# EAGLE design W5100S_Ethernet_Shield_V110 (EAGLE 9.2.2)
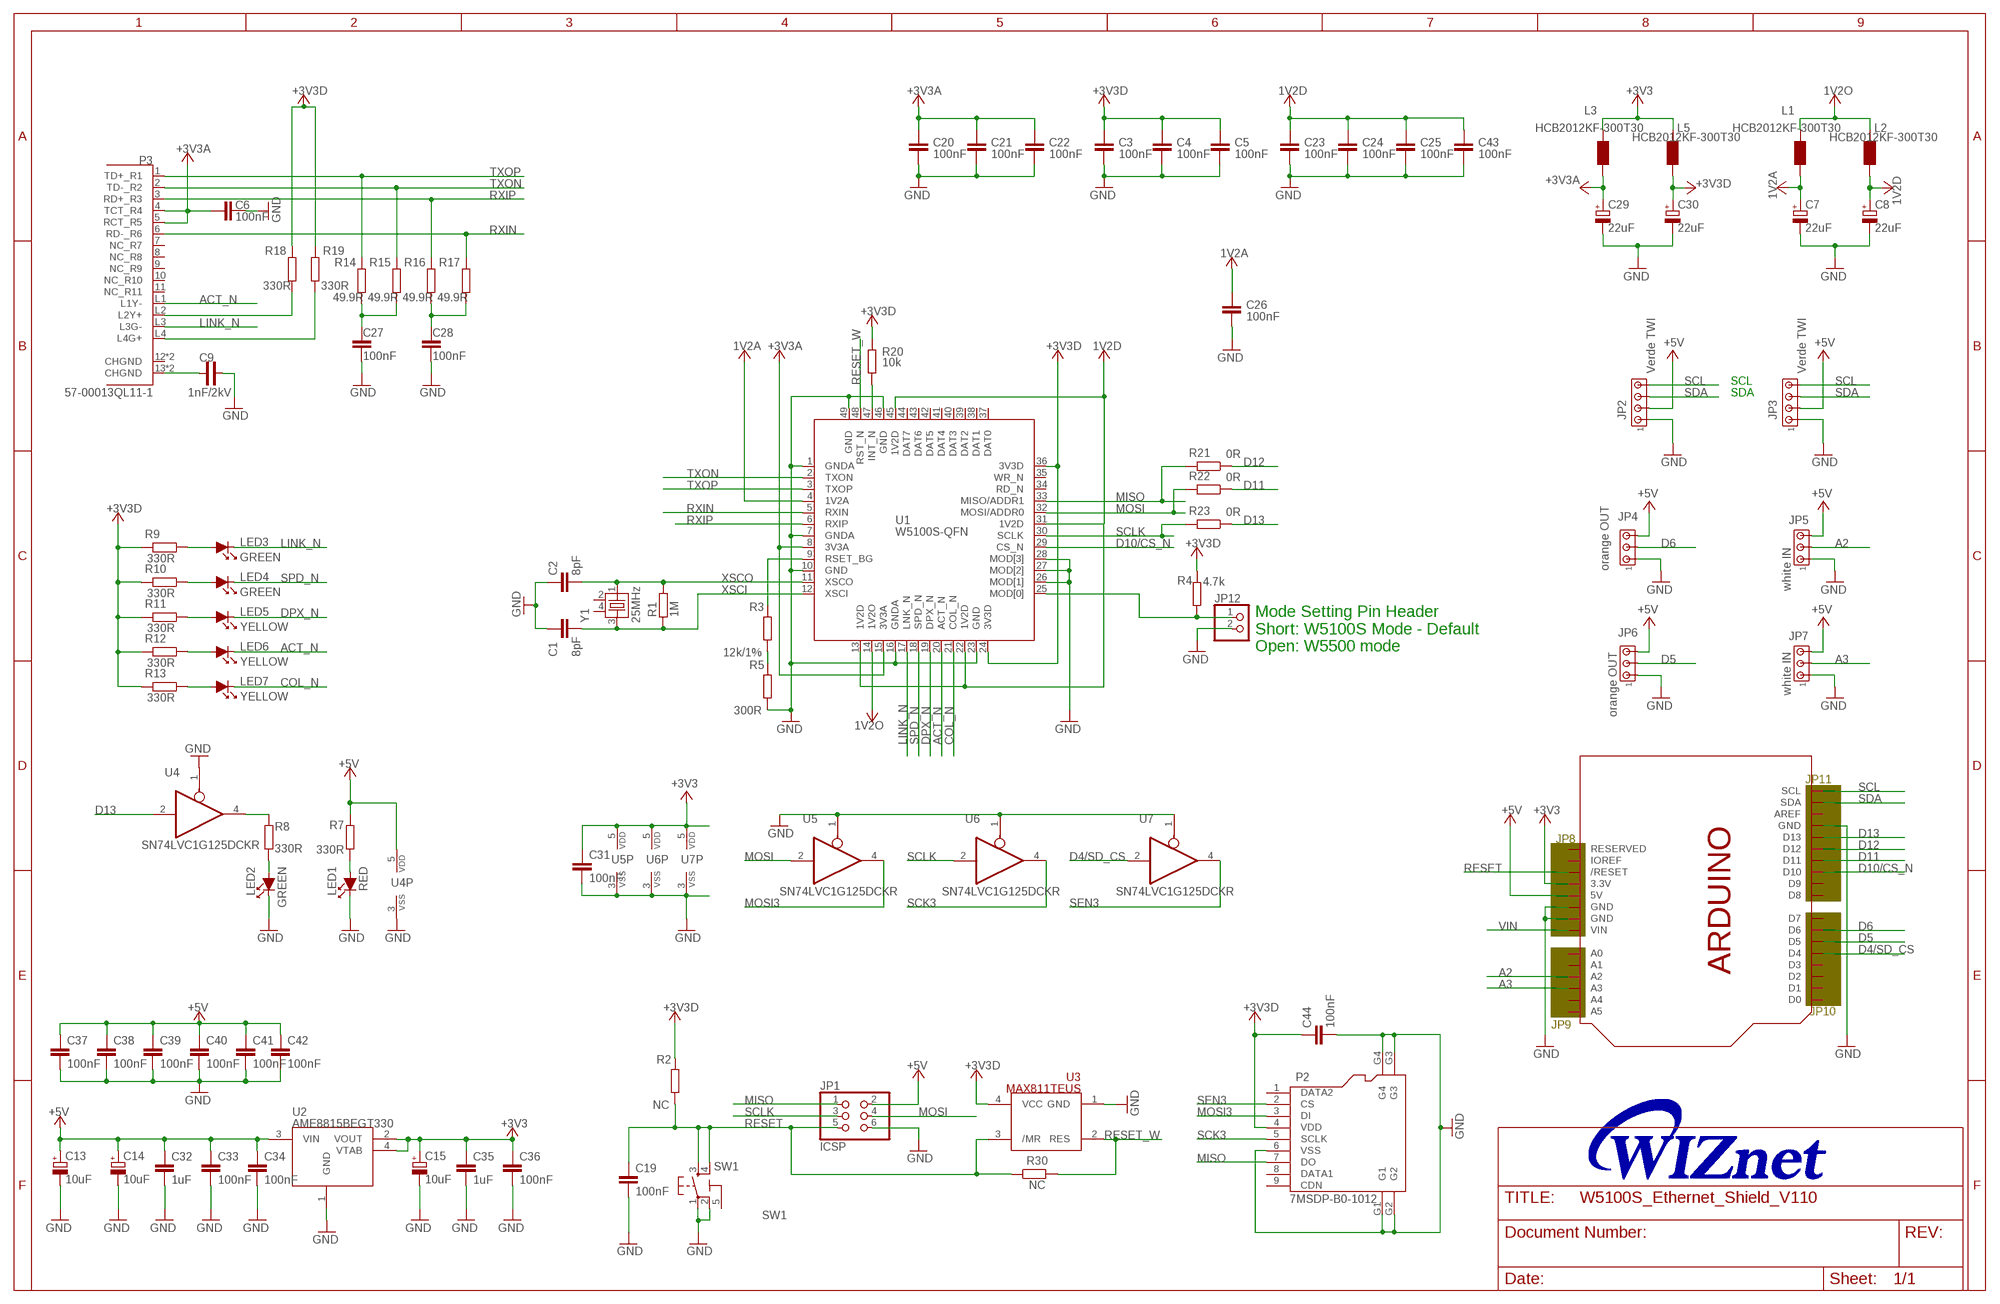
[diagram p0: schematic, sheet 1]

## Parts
C1  8pF  C-EU0603-RND  [C0603-ROUND]
C2  8pF  C-EU0603-RND  [C0603-ROUND]
C3  100nF  C-EU0603-RND  [C0603-ROUND]
C4  100nF  C-EU0603-RND  [C0603-ROUND]
C5  100nF  C-EU0603-RND  [C0603-ROUND]
C6  100nF  0142_10NF_0603  [C0603-ROUND@1]
C7  22uF  0474_TAJA475M016RNJ  [SMC_A]
C8  22uF  0474_TAJA475M016RNJ  [SMC_A]
C9  1nF/2kV  C-4520  [C-4520]
C13  10uF  0474_TAJA475M016RNJ  [SMC_A]
C14  10uF  0474_TAJA475M016RNJ  [SMC_A]
C15  10uF  0474_TAJA475M016RNJ  [SMC_A]
C19  100nF  0142_10NF_0603  [C0603-ROUND@1]
C20  100nF  C-EU0603-RND  [C0603-ROUND]
C21  100nF  C-EU0603-RND  [C0603-ROUND]
C22  100nF  C-EU0603-RND  [C0603-ROUND]
C23  100nF  C-EU0603-RND  [C0603-ROUND]
C24  100nF  C-EU0603-RND  [C0603-ROUND]
C25  100nF  C-EU0603-RND  [C0603-ROUND]
C26  100nF  C-EU0603-RND  [C0603-ROUND]
C27  100nF  0142_10NF_0603  [C0603-ROUND@1]
C28  100nF  0142_10NF_0603  [C0603-ROUND@1]
C29  22uF  0474_TAJA475M016RNJ  [SMC_A]
C30  22uF  0474_TAJA475M016RNJ  [SMC_A]
C31  100nF  0006_1UF_0603/GRM188R61E105KA12D  [C0603-ROUND]
C32  1uF  0142_10NF_0603  [C0603-ROUND@1]
C33  100nF  0142_10NF_0603  [C0603-ROUND@1]
C34  100nF  0142_10NF_0603  [C0603-ROUND@1]
C35  1uF  0142_10NF_0603  [C0603-ROUND@1]
C36  100nF  0142_10NF_0603  [C0603-ROUND@1]
C37  100nF  0142_10NF_0603  [C0603-ROUND@1]
C38  100nF  0142_10NF_0603  [C0603-ROUND@1]
C39  100nF  0142_10NF_0603  [C0603-ROUND@1]
C40  100nF  0142_10NF_0603  [C0603-ROUND@1]
C41  100nF  0142_10NF_0603  [C0603-ROUND@1]
C42  100nF  0142_10NF_0603  [C0603-ROUND@1]
C43  100nF  C-EU0603-RND  [C0603-ROUND]
C44  100nF  0006_1UF_0603/GRM188R61E105KA12D  [C0603-ROUND]
JP1  ICSP  0114_PH254-203DF118A00V  [2X03]
JP2  Verde TWI  1693_WA254-04S-632  [10X04MTA]
JP3  Verde TWI  1693_WA254-04S-632  [10X04MTA]
JP4  orange OUT  1696_WA254-03S-166  [10X03MTA]
JP5  white IN  1695_WA254-03S-IN  [10X03MTA]
JP6  orange OUT  0141_LHA-03-TS  [10X03MTA]
JP7  white IN  1695_WA254-03S-IN  [10X03MTA]
JP12  PINHD-1X2  [1X02]
L1  HCB2012KF-300T30  0001_BLM21PG300SN1D_/_MH2029-300Y  [0805]
L2  HCB2012KF-300T30  0001_BLM21PG300SN1D_/_MH2029-300Y  [0805]
L3  HCB2012KF-300T30  0001_BLM21PG300SN1D_/_MH2029-300Y  [0805]
L5  HCB2012KF-300T30  0001_BLM21PG300SN1D_/_MH2029-300Y  [0805]
LED1  RED  LED-1608  [LED-1608]
LED2  GREEN  LED-1608  [LED-1608]
LED3  GREEN  LED-1608  [LED-1608]
LED4  GREEN  LED-1608  [LED-1608]
LED5  YELLOW  LED-1608  [LED-1608]
LED6  YELLOW  LED-1608  [LED-1608]
LED7  YELLOW  LED-1608  [LED-1608]
P2  7MSDP-B0-1012  MICRO-SD-CARD-SOCKET-9P(ST-TF-003A)  [MICRO-SD9+4P-SMD-16.1X14.5X1.85MM]
P3  57-00013QL11-1  [57-00013QL11-1]
R1  1M  RESISTENZE_0026_100K_0603  [RESISTENZE_R0603-ROUND]
R2  NC  0028_CR0603JW103L  [R0603-ROUND]
R3  12k/1%  0028_CR0603JW103L  [R0603-ROUND]
R4  4.7k  0028_CR0603JW103L  [R0603-ROUND]
R5  300R  0028_CR0603JW103L  [R0603-ROUND]
R7  330R  RESISTENZE_0026_100K_0603  [RESISTENZE_R0603-ROUND]
R8  330R  RESISTENZE_0026_100K_0603  [RESISTENZE_R0603-ROUND]
R9  330R  0028_CR0603JW103L  [R0603-ROUND]
R10  330R  0028_CR0603JW103L  [R0603-ROUND]
R11  330R  0028_CR0603JW103L  [R0603-ROUND]
R12  330R  0028_CR0603JW103L  [R0603-ROUND]
R13  330R  0028_CR0603JW103L  [R0603-ROUND]
R14  49.9R  RESISTENZE_0026_100K_0603  [RESISTENZE_R0603-ROUND]
R15  49.9R  RESISTENZE_0026_100K_0603  [RESISTENZE_R0603-ROUND]
R16  49.9R  RESISTENZE_0026_100K_0603  [RESISTENZE_R0603-ROUND]
R17  49.9R  RESISTENZE_0026_100K_0603  [RESISTENZE_R0603-ROUND]
R18  330R  RESISTENZE_0026_100K_0603  [RESISTENZE_R0603-ROUND]
R19  330R  RESISTENZE_0026_100K_0603  [RESISTENZE_R0603-ROUND]
R20  10k  0028_CR0603JW103L  [R0603-ROUND]
R21  0R  0028_CR0603JW103L  [R0603-ROUND]
R22  0R  0028_CR0603JW103L  [R0603-ROUND]
R23  0R  0028_CR0603JW103L  [R0603-ROUND]
R30  NC  0028_CR0603JW103L  [R0603-ROUND]
SW1  SW1  0946_TS42031-160W-TR-7260  [TS42]
U1  W5100S-QFN  [W5100S-QFN]
U2  AME8815BEGT330  [SOT-223]
U3  MAX811TEUS  0035_CAT811TTBI-GT3  [SOT143]
U4  SN74LVC1G125DCKR  0040_SN74LVC1G125DCKR  [SC70-5]
U5  SN74LVC1G125DCKR  0040_SN74LVC1G125DCKR  [SC70-5]
U6  SN74LVC1G125DCKR  0040_SN74LVC1G125DCKR  [SC70-5]
U7  SN74LVC1G125DCKR  0040_SN74LVC1G125DCKR  [SC70-5]
U$4  ARDUINO_R3_ICSP_4  [ARDUINOR3_ICSP_4]
Y1  25MHz  XTAL3225  [XTAL3225]

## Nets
1V2A: C7.+ C26.2 L1.1 U1.4(1V2A)
1V2D: C8.+ C23.2 C24.2 C25.2 C43.2 L2.1 U1.13(1V2D) U1.22(1V2D) U1.31(1V2D) U1.45(1V2D)
1V2O: L1.2 L2.2 U1.14(1V2O)
+3V3 [power]: C15.+ C31.1 C35.1 C36.1 L3.2 L5.2 U2.2(VOUT) U2.4(VTAB) U5.5(VDD) U6.5(VDD) U7.5(VDD) U$4.3V(3.3V)
+3V3A [power]: C6.1 C20.2 C21.2 C22.2 C29.+ L3.1 P3.4(TCT_R4) P3.5(RCT_R5) U1.8(3V3A) U1.15(3V3A)
+3V3D: C3.2 C4.2 C5.2 C30.+ C44.1 L5.1 P2.4(VDD) R2.2 R4.1 R9.2 R10.2 R11.2 R12.2 R13.2 R18.1 R19.1 R20.2 U1.24(3V3D) U1.36(3V3D) U3.4(VCC)
+5V [power]: C13.+ C14.+ C32.1 C33.1 C34.1 C37.1 C38.1 C39.1 C40.1 C41.1 C42.1 JP1.2 JP2.2 JP3.2 JP4.3 JP5.3 JP6.3 JP7.3 R7.2 U2.3(VIN) U4.5(VDD) U$4.5V
A2: JP5.2 U$4.A2
A3: JP7.2 U$4.A3
ACT_N: LED6.K P3.L1(L1Y-) U1.20(ACT_N)
COL_N: LED7.K U1.21(COL_N)
D4/SD_CS: U7.2(I) U$4.D4
D5: JP6.2 U$4.D5
D6: JP4.2 U$4.D6
D10/CS_N: U1.29(CS_N) U$4.D10
D11: R22.1 U$4.D11
D12: R21.1 U$4.D12
D13: R23.1 U4.2(I) U$4.D13
DPX_N: LED5.K U1.19(DPX_N)
GND [gnd]: C1.1 C2.1 C3.1 C4.1 C5.1 C6.2 C7.- C8.- C9.2 C13.- C14.- C15.- C19.2 C20.1 C21.1 C22.1 C23.1 C24.1 C25.1 C26.1 C27.1 C28.1 C29.- C30.- C31.2 C32.2 C33.2 C34.2 C35.2 C36.2 C37.2 C38.2 C39.2 C40.2 C41.2 C42.2 C43.1 C44.2 JP1.6 JP2.1 JP3.1 JP4.1 JP5.1 JP6.1 JP7.1 JP12.2 LED1.K LED2.K P2.6(VSS) P2.G1 P2.G2 P2.G3 P2.G4 R5.1 SW1.1 SW1.2 U1.1(GNDA) U1.7(GNDA) U1.10(GND) U1.16(GNDA) U1.23(GND) U1.26(MOD[1]) U1.27(MOD[2]) U1.28(MOD[3]) U1.46(GND) U1.49(GND) U2.1(GND) U3.1(GND) U4.1(OE) U4.3(VSS) U5.1(OE) U5.3(VSS) U6.1(OE) U6.3(VSS) U7.1(OE) U7.3(VSS) U$4.GND U$4.GND@1(GND) U$4.GND@2(GND)
LINK_N: LED3.K P3.L3(L3G-) U1.17(LNK_N)
MISO: JP1.1 P2.7(DO) R21.2 U1.33(MISO/ADDR1)
MOSI: JP1.4 R22.2 U1.32(MOSI/ADDR0) U5.2(I)
MOSI3: P2.3(DI) U5.4(O)
N$1: LED3.A R9.1
N$2: P3.L2(L2Y+) R18.2
N$3: LED1.A R7.1
N$4: LED4.A R10.1
N$5: LED5.A R11.1
N$6: LED6.A R12.1
N$7: LED7.A R13.1
N$8: P3.L4(L4G+) R19.2
N$9: C9.1 P3.13(CHGND) P3.P$4(CHGND)
N$10: R3.1 R5.2
N$12: C27.2 R14.2 R15.2
N$13: R8.2 U4.4(O)
N$14: LED2.A R8.1
N$15: C28.2 R16.2 R17.2
N$16: R20.1 U1.47(INT_N)
N$17: JP12.1 R4.2 U1.25(MOD[0])
N$20: R3.2 U1.9(RSET_BG)
RESET: C19.1 JP1.5 R2.1 R30.1 SW1.3 SW1.4 U3.3(/MR) U$4.RESET(/RESET)
RESET_W: R30.2 U1.48(RST_N) U3.2(RES)
RXIN: P3.6(RD-_R6) R17.1 U1.5(RXIN)
RXIP: P3.3(RD+_R3) R16.1 U1.6(RXIP)
SCK3: P2.5(SCLK) U6.4(O)
SCL: JP2.4 JP3.4 U$4.SCL
SCLK: JP1.3 R23.2 U1.30(SCLK) U6.2(I)
SDA: JP2.3 JP3.3 U$4.SDA
SEN3: P2.2(CS) U7.4(O)
SPD_N: LED4.K U1.18(SPD_N)
TXON: P3.2(TD-_R2) R15.1 U1.2(TXON)
TXOP: P3.1(TD+_R1) R14.1 U1.3(TXOP)
VIN [gnd]: U$4.VIN
XSCI: C1.2 R1.1 U1.12(XSCI) Y1.3
XSCO: C2.2 R1.2 U1.11(XSCO) Y1.1
Unconnected: P2.1(DATA2) P2.8(DATA1) P2.9(CDN) P3.7(NC_R7) P3.8(NC_R8) P3.9(NC_R9) P3.10(NC_R10) P3.11(NC_R11) P3.12(CHGND) P3.P$3(CHGND) U1.34(RD_N) U1.35(WR_N) U1.37(DAT0) U1.38(DAT1) U1.39(DAT2) U1.40(DAT3) U1.41(DAT4) U1.42(DAT5) U1.43(DAT6) U1.44(DAT7) U$4.A0 U$4.A1 U$4.A4 U$4.A5 U$4.AREF U$4.D0 U$4.D1 U$4.D2 U$4.D3 U$4.D7 U$4.D8 U$4.D9 U$4.IOREF U$4.RESERVED Y1.2 Y1.4

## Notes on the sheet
- SCL
- SDA
- Mode Setting Pin Header
  Short: W5100S Mode - Default
  Open: W5500 mode
- JP11
- JP8
- JP10
- JP9

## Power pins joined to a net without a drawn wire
5-GND: SW1.5(5-GND)

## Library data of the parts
C1-C5 C20-C26 C43 = SmartPrj:C-EU: CAPACITOR, European symbol
C6 C19 C27 C28 C32-C42 = Condensatori:0142_10NF_0603: 10nF 0603; CASE: 0603; MONTHLY_USAGE: _____; PART_NUMBER: 10nF_0603; PRICE: _____; SUPPLIER: _____; TYPE: Condensatori; VALUE: 10nF
C7 C8 C13-C15 C29 C30 = Condensatori:0474_TAJA475M016RNJ: 4u7 tantalio Case A - testa gialla -Tantalio; CASE: CaseA_(1206); MONTHLY_USAGE: _____; PART_NUMBER: TAJA475M016RNJ; PRICE: _____; SUPPLIER: _____; TYPE: Condensatori; VALUE: 4u7
C9 = CAP:C-4520
C31 C44 = Condensatori:0006_1UF_0603/GRM188R61E105KA12D: 1uF 0603; CASE: 0603; MONTHLY_USAGE: 207014.16; PART_NUMBER: 1uF_0603/GRM188R61E105KA12D; PRICE: �_0.00; SUPPLIER: La_Tecnika_Due_s.r.l.; TYPE: Condensatori; VALUE: 1uF
JP1 = Connettori:0114_PH254-203DF118A00V: 3x2 M V h 8,5 mm p2,54; MONTHLY_USAGE: _____; PART_NUMBER: PH254-203DF118A00V; PRICE: _____; SUPPLIER: _____; TYPE: Connettori
JP2 JP3 = Connettori:1693_WA254-04S-632: 4x1 V Verde p 2,54 Serigrafato TWI; MONTHLY_USAGE: _____; PART_NUMBER: WA254-04S-632; PRICE: _____; SUPPLIER: _____; TYPE: Connettori; VALUE: WA254-04S-632
JP4 = Connettori:1696_WA254-03S-166: 3x1 Poli V Arancioni Serigrafati OUT; MONTHLY_USAGE: _____; PART_NUMBER: WA254-03S-166; PRICE: _____; SUPPLIER: _____; TYPE: Connettori; VALUE: WA254-03S-166
JP5 JP7 = Connettori:1695_WA254-03S-IN: 3x1 V Bianco P2,54 Serigrafati IN; MONTHLY_USAGE: _____; PART_NUMBER: WA254-03S-IN; PRICE: _____; SUPPLIER: _____; TYPE: Connettori; VALUE: WA254-03S-IN
JP6 = Connettori:0141_LHA-03-TS: 3x1 V Bianco P2,54; MONTHLY_USAGE: _____; PART_NUMBER: LHA-03-TS; PRICE: _____; SUPPLIER: _____; TYPE: Connettori; VALUE: LHA-03-TS
JP12 = PinHeader:PINHD-1X2: PIN HEADER
L1-L3 L5 = Protezione:0001_BLM21PG300SN1D_/_MH2029-300Y: BLM21; MONTHLY_USAGE: _____; PART_NUMBER: BLM21PG300SN1D_/_MH2029-300Y; PRICE: _____; SUPPLIER: _____; TYPE: Protezione; VALUE: MH2029-300Y
LED1-LED7 = DIODE:LED-1608
P2 = Seeed-OPL-Connector:MICRO-SD-CARD-SOCKET-9P(ST-TF-003A): 320090000; MPN: ST-TF-003A; VALUE: ST-TF-003A
P3 = WIZnet:57-00013QL11-1
R1 R7 R8 R14-R19 = Arduino-M0-V1:RESISTENZE_0026_100K_0603: 100K 0603; CASE: 0603; MONTHLY_USAGE: _____; PART_NUMBER: 100K_0603; PRICE: _____; SUPPLIER: _____; TYPE: Resistenze; VALUE: 100k
R2-R5 R9-R13 R21-R23 R30 = Resistenze:0028_CR0603JW103L: 10K 0603; CASE: 0603; MONTHLY_USAGE: _____; PART_NUMBER: CR0603JW103L; PRICE: _____; SUPPLIER: _____; TYPE: Resistenze; VALUE: 10k
R20 = Resistenze:0028_CR0603JW103L: 10K 0603; CASE: 0603; MONTHLY_USAGE: _____; PART_NUMBER: CR0603JW103L; PRICE: _____; SUPPLIER: _____; TYPE: Resistenze
SW1 = Switches:0946_TS42031-160W-TR-7260: Pushbutton 6x6 Smd - White; MONTHLY_USAGE: _____; PART_NUMBER: IT-1157AHNP-160G-G_GTR; PRICE: _____; SUPPLIER: _____; TYPE: Switches; VALUE: TS42
U1 = WIZnet:W5100S-QFN
U2 = RECULATOR:AME8815BEGT330
U3 = Circuito Integrato:0035_CAT811TTBI-GT3: 4-Pin Microprocessor Power Supply Supervisors- Reset Controller CAT811TTBI-GT3; CASE: SOT143-4; MONTHLY_USAGE: _____; PART_NUMBER: CAT811TTBI-GT3; PRICE: _____; SUPPLIER: _____; TYPE: Circuito_Integrato; VALUE: CAT811TTBI-GT3
U4-U7 = Circuito Integrato:0040_SN74LVC1G125DCKR: Single bus buffer with 3-state output; CASE: SC70; MONTHLY_USAGE: _____; PART_NUMBER: SN74LVC1G125DCKR; PRICE: _____; SPICEPREFIX: U; SUPPLIER: _____; TYPE: Circuito_Integrato; VALUE: 74LVC1G125DCKR
U$4 = Arduino:ARDUINO_R3_ICSP_4
Y1 = X-TAL:XTAL3225

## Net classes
1 power: width 0.254 mm, drill 0.61 mm, clearance 0.203 mm
2 gnd: width 0.254 mm, drill 0.3 mm, clearance 0.127 mm

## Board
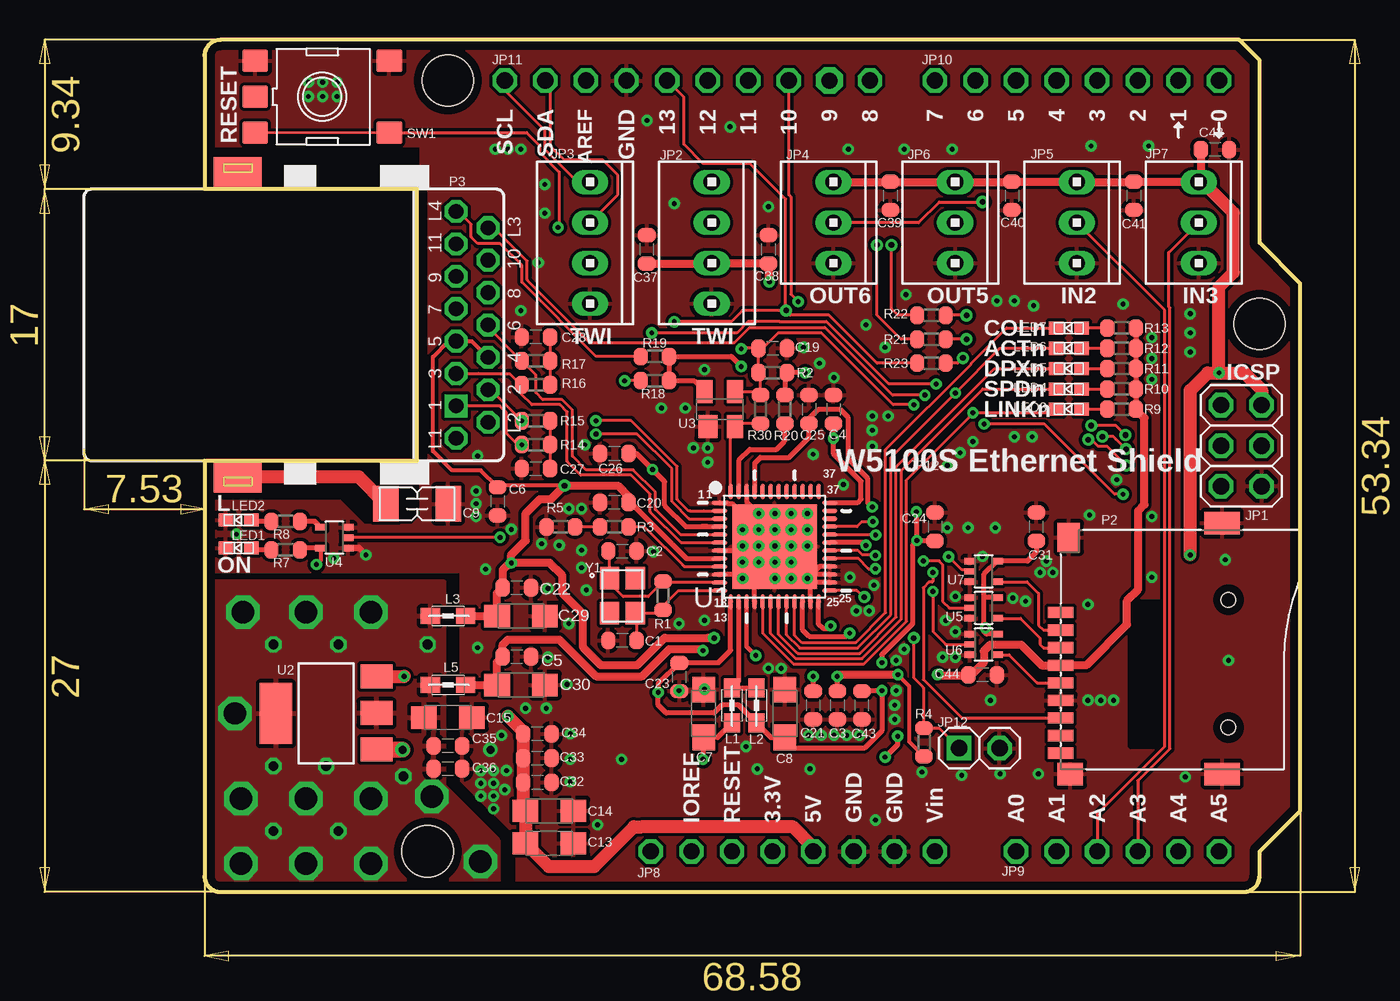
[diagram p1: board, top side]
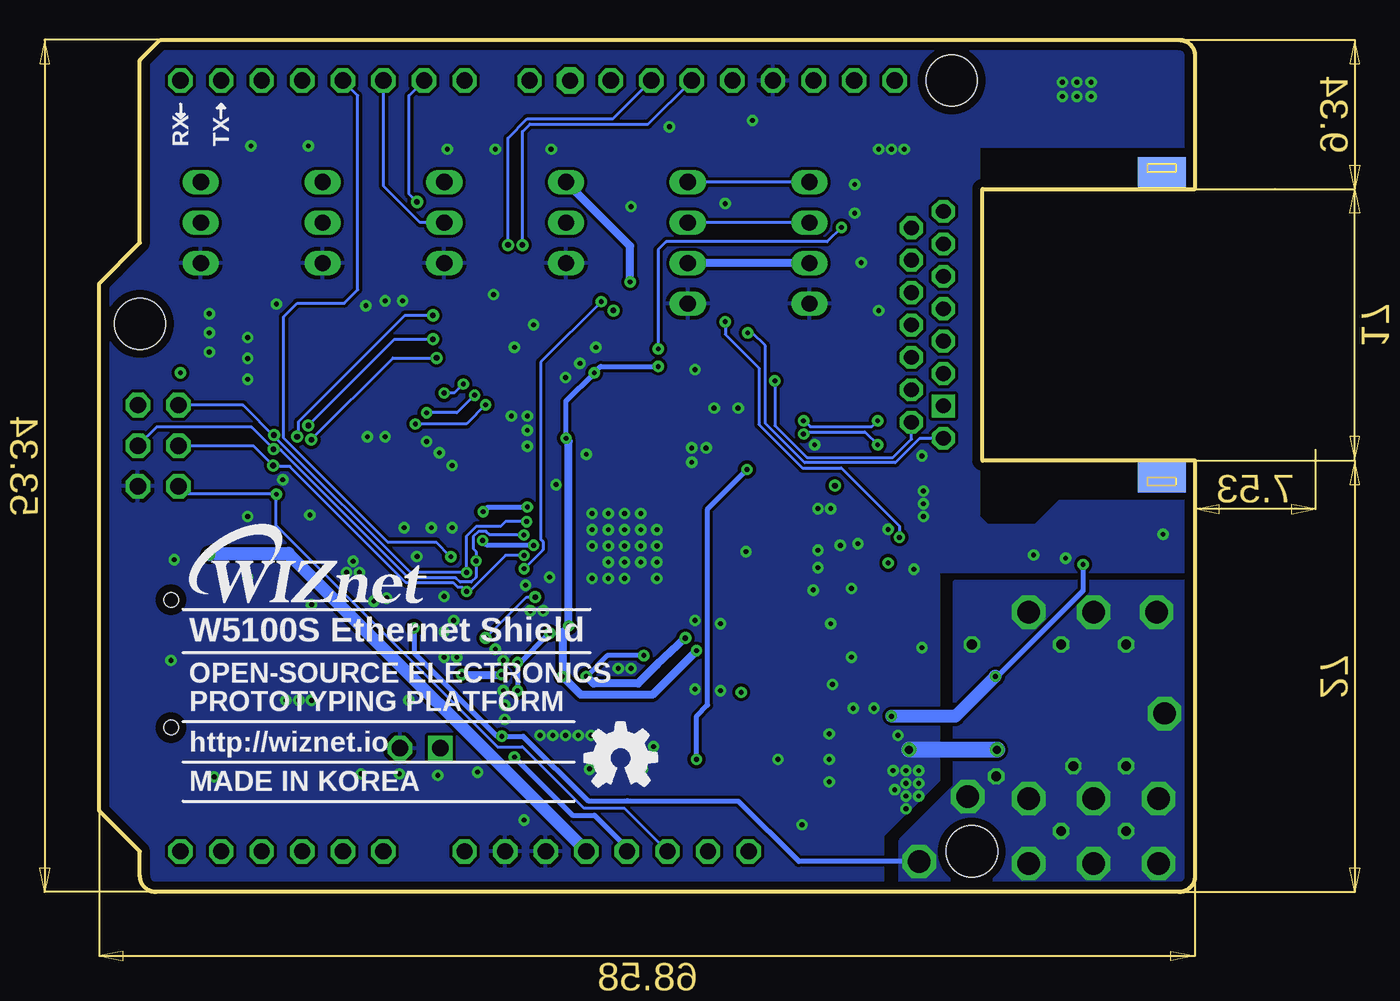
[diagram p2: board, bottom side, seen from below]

Size 82.6 x 57.64 mm. Coordinates in mm from the lower left corner, seen from the top.
Outline: 76.34,6.84 78.88,9.38 78.88,42.4 76.34,44.94 76.34,56.37 75.07,57.64 11.3,57.64 arc90 10.3,56.64 10.3,48.3 23.6,48.3 23.6,31.3 10.3,31.3 10.3,5.3 arc90 11.3,4.3 75.34,4.3 arc90 76.34,5.3 76.34,6.84
Copper layers (1*16): Top 0.035mm / dielectric 1.5mm / Bottom 0.035mm
Design rules "default *": minimum track width 6mil, minimum drill 0.2mm, track to track 5mil, track to pad 5mil, pad to pad 5mil, via to via 5mil, smd to smd 4mil, copper to edge 20mil, drill to drill 10mil, minimum pad ring 10mil, minimum via ring 8mil, stop-mask expansion 1mil, vias tented up to drill 15mil, thermal gap 10mil

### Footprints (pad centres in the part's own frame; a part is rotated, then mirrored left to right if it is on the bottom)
C0603-ROUND = smd 0.898 x 1.1: 1 -0.889,0; 2 0.889,0
C0603-ROUND@1 = smd 0.898 x 1.1: 1 -0.889,0; 2 0.889,0
SMC_A = smd 1.6 x 1.4: + -1.5,0; - 1.5,0
C-4520 = smd 1.6 x 2.2: 1 -1.95,0; 2 1.95,0
2X03 = drill 1.016 pad 1.55 octagon: 1 -2.54,-1.27; 2 -2.54,1.27; 3 0,-1.27; 4 0,1.27; 5 2.54,-1.27; 6 2.54,1.27
10X04MTA = drill 1.016 long: 1 3.81,0; 2 1.27,0; 3 -1.27,0; 4 -3.81,0
10X03MTA = drill 1.016 long: 1 2.54,0; 2 0,0; 3 -2.54,0
1X02 = drill 1.016 square: 1 -1.27,0 | drill 1.016 octagon: 2 1.27,0
0805 = smd 1.2 x 1: 1 -1.1,0; 2 1.1,0
LED-1608 = smd 0.89 x 0.82: A -0.8,0; K 0.8,0
MICRO-SD9+4P-SMD-16.1X14.5X1.85MM = smd 1.6 x 0.7: 1 0,2.25; 2 0,1.15; 3 0,0.05; 4 0,-1.05; 5 0,-2.15; 6 0,-3.25; 7 0,-4.35; 8 0,-5.45; 9 0,-6.55 | smd 1.6 x 1.4: G1 0.6,-7.85 | smd 2.2 x 1.4: G2 10.1,-7.85; G3 10.1,7.85 | smd 1.4 x 1.8: G4 0.5,6.95 | hole 0.9: 10.5,-4.95; 10.5,3.05
57-00013QL11-1 = drill 0.914 square: 1 5.075,10.15 | drill 0.914 octagon: 2 4.065,12.15; 3 3.045,10.15; 4 2.035,12.15; 5 1.015,10.15; 6 0.005,12.15; 7 -1.015,10.15; 8 -2.025,12.15; 9 -3.045,10.15; 10 -4.055,12.15; 11 -5.075,10.15; L1 7.105,10.15; L2 6.095,12.15; L3 -6.085,12.15; L4 -7.105,10.15 | smd 2 x 3: 12 -9.5,-3.51; 13 9.5,-3.51 | smd 2 x 3 bottom: P$3 -9.5,-3.51; P$4 9.5,-3.51
RESISTENZE_R0603-ROUND = smd 0.898 x 1.1: 1 -0.889,0; 2 0.889,0
R0603-ROUND = smd 0.898 x 1.1: 1 -0.889,0; 2 0.889,0
TS42 = smd 1.6 x 1.4: 1 -4.2,2.25; 2 4.2,2.25; 3 -4.2,-2.25; 4 4.2,-2.25; 5 -4.2,0
W5100S-QFN = smd 0.95 x 0.25: 1 -3.45,2.75; 2 -3.45,2.25; 3 -3.45,1.75; 4 -3.45,1.25; 5 -3.45,0.75; 6 -3.45,0.25; 7 -3.45,-0.25; 8 -3.45,-0.75; 9 -3.45,-1.25; 10 -3.45,-1.75; 11 -3.45,-2.25; 12 -3.45,-2.75; 25 3.45,-2.75; 26 3.45,-2.25; 27 3.45,-1.75; 28 3.45,-1.25; 29 3.45,-0.75; 30 3.45,-0.25; 31 3.45,0.25; 32 3.45,0.75; 33 3.45,1.25; 34 3.45,1.75; 35 3.45,2.25; 36 3.45,2.75 | smd 0.25 x 0.95: 13 -2.75,-3.45; 14 -2.25,-3.45; 15 -1.75,-3.45; 16 -1.25,-3.45; 17 -0.75,-3.45; 18 -0.25,-3.45; 19 0.25,-3.45; 20 0.75,-3.45; 21 1.25,-3.45; 22 1.75,-3.45; 23 2.25,-3.45; 24 2.75,-3.45; 37 2.75,3.45; 38 2.25,3.45; 39 1.75,3.45; 40 1.25,3.45; 41 0.75,3.45; 42 0.25,3.45; 43 -0.25,3.45; 44 -0.75,3.45; 45 -1.25,3.45; 46 -1.75,3.45; 47 -2.25,3.45; 48 -2.75,3.45 | smd 5.3 x 5.3: 49 0,0
SOT-223 = smd 1.499 x 2.007: 1 -2.261,-3.15; 2 0.025,-3.15; 3 2.311,-3.15 | smd 3.81 x 2.007: 4 0,3.15
SOT143 = smd 1.2 x 1.44: 1 -0.75,-1.1 | smd 1 x 1.44: 2 0.95,-1.1; 3 0.95,1.1; 4 -0.95,1.1
SC70-5 = smd 0.4 x 0.7: 1 -0.65,-0.85; 2 0,-0.85; 3 0.65,-0.85; 4 0.65,0.85; 5 -0.65,0.85
ARDUINOR3_ICSP_4 = drill 1.016 octagon: 3V 35.56,2.54; 5V 38.1,2.54; A0 50.8,2.54; A1 53.34,2.54; A2 55.88,2.54; A3 58.42,2.54; A4 60.96,2.54; A5 63.5,2.54; AREF 23.876,50.8; D0 63.5,50.8; D1 60.96,50.8; D2 58.42,50.8; D3 55.88,50.8; D4 53.34,50.8; D5 50.8,50.8; D6 48.26,50.8; D7 45.72,50.8; D8 41.656,50.8; D10 36.576,50.8; D11 34.036,50.8; D12 31.496,50.8; D13 28.956,50.8; GND 26.416,50.8; GND@1 43.18,2.54; GND@2 40.64,2.54; IOREF 30.48,2.54; RESERVED 27.94,2.54; RESET 33.02,2.54; SCL 18.796,50.8; SDA 21.336,50.8; VIN 45.72,2.54 | drill 1 pad 1.676 octagon: D9 39.116,50.8 | hole 3.2: 66.04,35.56; 15.24,50.8; 13.97,2.54
XTAL3225 = smd 1.4 x 1.2: 1 -1.1,-0.8; 2 1.1,-0.8; 3 1.1,0.8; 4 -1.1,0.8

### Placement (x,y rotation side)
C1  36.46,20.05 0 top
C2  36.46,25.64 180 top
C3  49.92,15.98 90 top
C4  49.67,34.53 270 top
C5  29.86,19.03 180 top
C6  28.65,28.75 270 top
C7  41.54,15.48 90 top
C8  46.62,15.48 90 top
C9  23.6,28.6 0 top
C13  31.89,7.35 0 top
C14  31.89,9.38 0 top
C15  25.54,15.22 0 top
C19  45.86,38.34 0 top
C20  35.95,28.68 0 top
C21  48.4,15.98 90 top
C22  29.86,23.35 180 top
C23  40.02,17.76 90 top
C24  56.02,27.16 270 top
C25  48.15,34.53 270 top
C26  35.95,31.74 0 top
C27  31.05,30.8 0 top
C28  31.05,39.05 0 top
C29  30.11,21.57 0 top
C30  30.11,17.25 0 top
C31  62.37,27.16 90 top
C32  31.13,11.16 0 top
C33  31.13,12.68 0 top
C34  31.13,14.21 0 top
C35  25.54,13.44 0 top
C36  25.54,12.02 0 top
C37  37.99,44.53 90 top
C38  45.61,44.53 90 top
C39  53.23,47.89 270 top
C40  60.85,47.89 270 top
C41  68.47,47.89 270 top
C42  73.55,50.78 0 top
C43  51.45,15.98 90 top
C44  59,17.9 0 top
JP1  75.2,32.24 270 top
JP2  42.05,44.94 270 top
JP3  34.43,44.94 270 top
JP4  49.67,46.21 270 top
JP5  64.91,46.21 270 top
JP6  57.29,46.21 270 top
JP7  72.53,46.21 270 top
JP12  58.8,13.3 0 top
L1  43.32,15.98 90 top
L2  44.84,15.98 90 top
L3  25.54,21.57 180 top
L5  25.54,17.25 180 top
LED1  12.43,25.84 180 top
LED2  12.43,27.58 180 top
LED3  64.4,34.53 180 top
LED4  64.4,35.8 180 top
LED5  64.4,37.07 180 top
LED6  64.4,38.34 180 top
LED7  64.4,39.61 180 top
P2  63.89,19.54 0 top
P3  15.9,39.8 270 top
R1  39,22.84 90 top
R2  45.86,36.81 0 top
R3  35.95,27.16 0 top
R4  55.34,13.67 90 top
R5  32.6,27.16 0 top
R7  15.38,25.72 0 top
R8  15.38,27.5 0 top
R9  67.7,34.53 0 top
R10  67.7,35.8 0 top
R11  67.7,37.07 0 top
R12  67.7,38.34 0 top
R13  67.7,39.61 0 top
R14  31.05,32.3 0 top
R15  31.05,33.8 0 top
R16  31.05,36.05 0 top
R17  31.05,37.55 0 top
R18  38.49,36.3 180 top
R19  38.49,37.83 180 top
R20  46.62,34.53 90 top
R21  55.8,38.9 0 top
R22  55.8,40.4 0 top
R23  55.8,37.4 0 top
R30  45.1,34.53 270 top
SW1  17.67,54.08 0 top
U1  45.99,25.92 0 top
U2  17.92,15.48 90 top
U3  42.56,34.53 0 top
U4  18.43,26.48 90 top
U5  59.07,22.08 270 top
U6  59.07,19.79 270 top
U7  59.07,24.37 270 top
U$3  [WIZNET2-LOGO]  74.15,21.21 0 bottom
U$4  10.3,4.3 0 top
U$5  [OSHP-LOGO]  49.3,10.3 0 bottom
Y1  36.46,22.84 270 top

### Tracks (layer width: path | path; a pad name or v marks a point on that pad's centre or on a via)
1V2A  (via drill 0.3)
  Top 0.3: L1.1 42.41,13.98 C7.+ 41.54,12.64 v41.5,12.6 | 41.78,27.16 41.41,27.16 | v38.34,30.74 38.24,30.84 | v38.34,30.74 39.1,29.98 39.1,28.5 40.44,27.16 41.78,27.16 | v38.34,30.74 37.34,31.74 C26.2 | 41.78,27.16 U1.4
  Bottom 0.3: v38.34,30.74 40.8,28.28 40.8,16 41.5,15.3 v41.5,12.6 41.5,12.5
1V2D  (via drill 0.3)
  Top 0.3: C8.+ 45.75,13.98 L2.1 43.73,16 42.7,16 42.2,15.5 39.2,15.5 38.7,16 v38.7,16.8 38.7,17.33 C23.2 42.45,18.65 43.24,19.44 U1.13 | 51.53,26.16 v51.7,26 51.53,26.16 | v54.9,26.3 55.99,26.3 C24.2 | v50.69,20.5 50.48,20.3 48.15,20.3 47.74,20.71 U1.22 | C43.2 51.47,16.9 v52.7,16.9 52.7,14.4 51.6,13.3 47.3,13.3 C8.+ | C8.+ 46.9,13.7 | v54.9,26.3 54.62,26.02 54.62,21.09 52.7,19.17 v52.7,18.66 | v54.9,26.3 54.9,28.06 v54.86,28.1 | v52.1,28.4 51.83,28.67 51.83,30.18 50.6,31.4 50.6,34 50.1,34.5 48.7,34.5 48.15,33.95 C25.2 48.15,32.75 46.9,31.5 45.1,31.5 44.74,31.14 U1.45 | 51.53,26.16 U1.31
  Bottom 0.3: v51.7,26 54.6,26 v54.9,26.3 | v50.69,20.5 52.7,18.49 | 52.7,18.49 v52.7,16.9 | v52.7,18.66 52.7,18.49 | v54.86,28.1 54.56,28.4 v52.1,28.4
1V2O
  Top 0.3: L2.2 L1.2 43.74,17.5 U1.14
+3V3  (via drill 0.3, 0.61, 1.4)
  Top 0.3: U6.5 59.26,20.44 59.1,20.6 59.1,20.76 | 59.1,20.76 59.1,22.8 | 59.1,22.8 59.1,24.2 U7.5 61.82,25.02 62.37,25.57 C31.1 | U5.5 59.17,22.73 59.1,22.8 | 59.1,20.76 v59.17,20.84 | v53.69,14.05 53.69,13.52 v52.9,12.74
  Bottom 0.254: U$4.3V 45.86,7.06
  Bottom 0.3: v59.17,20.84 59.17,19.25 53.97,14.05 v53.69,14.05 52.35,14.05 48.31,10.01 45.84,10.01 45.84,10 38.9,10 35.11,6.21 v27.57,6.21 | v52.9,12.74 49.26,9.1 47.9,9.1 45.86,7.06
  other vias: 14.62,12.17 17.92,12.17 16.65,10.14 20.71,10.14 14.62,8.11 18.68,8.11 12.59,10.14 16.65,6.08 20.71,6.08 12.59,6.08 22.75,11.54 24.52,10.27 12.21,15.48 12.21,15.48 12.71,21.83 16.65,21.83 14.62,19.79 18.68,19.79 24.27,19.79 20.71,21.83
  pour Top (isolate 0.2): 10.3,4.3 28.7,4.3 28.7,7.5 26.7,9.5 25.3,10.9 25.3,11.3 25.3,14.7 25.3,21.1 25.3,23.7 10.3,23.7
  pour Bottom (isolate 0.2): 10.3,4.1 28.7,4.1 28.7,7.5 25.3,10.9 25.3,23.7 10.3,23.7
+3V3A  (via drill 0.3, 0.35)
  Top 0.254: v32.84,29.74 28.75,29.74 C6.1 27.59,30.7 25.8,30.7 24.6,31.9 24.6,37.8 25.59,38.78 P3.5 27.03,38.78 P3.4
  Top 0.29: v44.8,19.1 44.24,19.66 U1.15
  Top 0.3: 39.56,26.08 | 39.56,26.08 40.48,25.16 U1.8 | v48.4,17.8 C21.2 | C20.2 36.96,28.68 39.56,26.08
  Top 0.5: L3.1 C29.+ 28.61,22.99 C22.2 28.97,24.47 29.4,24.9 v29.5,24.9 | 32.8,29.7 v32.84,29.74 | v32.84,29.74 36.17,29.74 36.84,29.07 C20.2 | v42.2,20.2 41.84,20.2 41.83,20.21 39.11,20.21 37.4,18.5 35.1,18.5 34,19.6 34,21.7 32.7,23 32.7,24.1 31.9,24.9 v29.5,24.9 | v29.5,24.9 29.5,25.4 30.4,26.3 30.4,28 31.3,28.9 32,28.9 v32.84,29.74
  Bottom 0.3: v44.8,19.1 47.1,19.1 v48.4,17.8
  Bottom 0.5: v42.2,20.2 44,18.5 45.16,17.34 47.94,17.34 v48.4,17.8
+3V3D  (via drill 0.3)
  Top 0.254: v53.7,17.9 54.4,17.2 54.4,13.72 R4.1
  Top 0.3: C4.2 v49.67,32.7 49.67,31.73 51.4,30 51.4,28.9 51.17,28.66 U1.36 | v49.9,17.8 49.9,16.9 C3.2 | R13.2 R12.2 R11.2 R10.2 R9.2 | R20.2 46.62,36.68 R2.2 47.89,36.81 v47.9,36.8 | v49.5,20.96 49.34,20.8 49,20.8 48.74,21.06 U1.24 | v43.9,37.2 43.27,37.83 R19.1 R18.1 40.93,36.3 U3.4
  Top 0.5: L5.1 C30.+ 28.61,18.68 C5.2 28.97,19.77 29.3,20.1 32.51,20.1 34.81,17.8 37.69,17.8 39.39,19.5 41.4,19.5 v41.5,19.4 | 49.94,17.84 v49.9,17.8 50,17.9 v53.7,17.9 | v56.2,17.9 56.26,17.84 58.05,17.84 C44.1 58.31,17.9 59.07,18.67 59.07,19.38 59.48,19.79 61.41,19.79 62.71,18.49 P2.4 65.49,18.49 68.04,21.04 68.04,22.54 68.74,23.24 68.74,28.16 69.14,28.56 69.14,33.98 R9.2
  Bottom 0.3: v49.67,32.7 49.67,35.03 v47.9,36.8 47.5,37.2 v43.9,37.2
  Bottom 0.5: v56.2,17.9 v53.7,17.9 | v49.67,32.7 49.5,32.53 v49.5,20.96 49.9,20.56 v49.9,17.8 48.74,16.64 44.26,16.64 v41.5,19.4
+5V  (via drill 0.3)
  Top 0.254: U4.5 17.58,25.08 v17.3,24.8 | U$4.5V 48.4,7.1
  Top 0.3: C14.+ | U4.5 16.38,25.83 R7.2
  Top 0.5: C34.1 | 37.96,43.67 C37.1 42.02,43.64 JP2.2 45.58,43.67 C38.1 45.61,42.55 v45.66,42.5 | C42.1 72.66,48.88 72.56,48.78 | 72.56,48.78 JP7.3 | JP4.3 53.2,48.75 C39.1 53.25,48.75 JP6.3 60.82,48.75 C40.1 64.88,48.78 JP5.3 68.44,48.75 C41.1 72.56,48.78
  Top 0.8: U2.3 22.79,17.79 v22.8,17.8 | v29.3,15.3 30.23,14.37 C34.1 | C34.1 C33.1 C32.1 30.24,9.53 C14.+ | C14.+ C13.+ 31.84,5.9 34.7,5.9 37.18,8.38 37.69,8.38 37.7,8.4 47.1,8.4 48.4,7.1 | v72,25.4 72,35.7 73.1,36.8 v73.8,36.8 | v73.8,36.8 75.4,36.8 76.47,35.73 JP1.2 | v73.8,36.8 73.8,42.17 74.71,43.08 74.71,46.83 72.66,48.88
  Bottom 0.3: v22.8,17.8 22.66,17.8 17.3,23.16 v17.3,24.8
  Bottom 0.5: JP3.2 JP2.2 | v45.66,42.5 45.66,44.74 JP4.3
  Bottom 0.8: v22.8,17.8 25.3,15.3 v29.3,15.3 | v72,25.4 71.7,25.5 67.06,25.5 U$4.5V
A2
  Top 0.2: JP5.2 70.4,40.72 70.4,13.41 66.18,9.18 U$4.A2
A3
  Top 0.2: JP7.2 70.65,44.33 70.65,40.93 70.73,40.85 70.73,13.27 68.72,11.26 U$4.A3
ACT_N  (via drill 0.3)
  Top 0.2: LED6.K 60.1,38.34 v57.3,35.54 53.26,31.5 53.26,21.65 51.18,19.57 47.56,19.57 46.74,20.4 U1.20 | v56.1,36.1 53.13,36.1 49.22,40.02 46.3,40.02 | v38.3,39.3 43.62,39.3 44.33,40.01 44.33,40.02
  Top 0.203: 46.3,40.02 44.33,40.02
  Bottom 0.2: v56.1,36.1 56.66,35.54 v57.3,35.54 | P3.L1 27.54,32.7 29.07,31.17 34.73,31.17 37.2,33.64 37.2,38.5 38,39.3 v38.3,39.3
COL_N
  Top 0.2: LED7.K 60.51,39.61 58.3,37.4 58.3,37.36 52.93,31.99 52.93,21.79 51.05,19.9 47.7,19.9 47.24,20.36 U1.21
D4/SD_CS  (via drill 0.3)
  Top 0.2: U7.2 58.12,24.46 57.72,24.46 56.9,25.28 v56.88,25.28
  Bottom 0.2: v56.88,25.28 57.8,26.2 60.84,26.2 67.34,32.71 67.34,40.3 66.5,41.15 63.55,41.15 62.7,42 62.7,54.16 U$4.D4
D5
  Bottom 0.2: JP6.2 58.81,46.21 61.1,48.5 U$4.D5
D6  (via drill 0.35)
  Top 0.2: v59,47.5 56.3,47.5 55,46.2 49.68,46.2 JP4.2
  Bottom 0.2: v59,47.5 59.5,48 59.5,54.16 U$4.D6
D10/CS_N  (via drill 0.3)
  Top 0.2: v52.3,24.54 51.86,24.54 51.23,25.16 U1.29 | v47.46,41.26 47,41.71 47,47.81 46.88,47.94 U$4.D10
  Bottom 0.2: v52.3,24.54 51.12,25.72 51.12,26.24 51.26,26.38 51.26,37.46 v47.46,41.26
D11  (via drill 0.35)
  Top 0.2: R22.1 53.7,40.4 53.3,40.8 v53.3,44.8
  Bottom 0.2: v53.3,44.8 53.3,51.5 52.1,52.7 46.74,52.7 U$4.D11
D12  (via drill 0.35)
  Top 0.2: R21.1 53.9,38.9 52.4,40.4 v52.4,44.8
  Bottom 0.2: v52.4,44.8 52.4,51.9 51.93,52.37 44.52,52.37 U$4.D12
D13  (via drill 0.3, 0.35)
  Top 0.2: U4.2 19.26,26.5 19.1,26.5 28.6,26.5 v28.8,26.5 | 46.68,40.72 46.68,40.8 | 46.68,40.8 46.68,47.68 44.46,49.9 41.5,49.9 40.3,51.1 40.3,54.06 U$4.D13 | R23.1 52.4,37.4 49.4,40.4 46.96,40.4 46.73,40.63 | 46.73,40.63 46.68,40.68 46.68,40.8 | v39.7,40 39.71,40.01 43.27,40.01 43.96,40.7 v46.7,40.7 46.7,40.66 46.73,40.63
  Bottom 0.2: v39.7,40 39.7,39.2 37.6,37.1 37.6,33.57 34.87,30.85 32.45,30.85 28.8,27.2 v28.8,26.5
DPX_N
  Top 0.2: LED5.K 59.75,37.07 53.59,30.9 53.59,21.52 51.32,19.25 47.43,19.25 46.24,20.44 U1.19
GND  (via drill 0.3, 0.5)
  Top 0.3: U1.16 44.74,24.69 v45,24.95 | 43.52,24.18 43.77,23.93 v43.98,23.93 43.74,24.17 U1.10 | U1.23 48.24,23.54 | 48.24,23.54 48.24,23.74 v48.05,23.93 48.28,24.16 | U1.26 48.36,23.66 48.24,23.54 | U1.28 48.78,24.66 48.28,24.16 | U1.27 48.28,24.16 | U1.46 44.24,28.76 v45,28 44.72,27.72 44.21,27.72 43.31,28.61 43.07,28.61 43.02,28.66 U1.1 | U1.7 43.68,25.66 v43.98,25.96
  Top 0.406: U4.1 19.97,25.83 v20.4,25.4
  Top 1: U2.1 22.69,13.21 v22.7,13.2
  Bottom 1: v22.7,13.2 v28.2,13.2
  other vias: 52.1,32.2 38.4,25.6 45.6,18.3 40,16.9 48.1,14.1 48.9,14.1 49.7,14.1 50.5,14.1 51.3,14.1 46.4,18.3 59,25.3 57.3,22.8 57.3,20.6 57.3,19 56.7,21.3 56.5,19 53.6,18.8 54.1,19.5 53.6,16.9 53.5,16 53.5,15.1 57.7,11.6 59.5,16.3 55.2,11.8 52.3,8.8 56.8,27.1 58.1,27.1 62.6,24.3 65.7,27.9 69.6,27.8 69.6,24 65.6,22.3 27.6,11.9 28.4,11.9 29.2,11.9 28.4,9.5 28.4,11.1 27.6,11.1 27.6,10.3 28.4,10.3 29.1,10.7 28.9,14.1 33,17.3 31.8,19 31.7,15.8 33.1,21.1 31.8,23.3 27.4,19.6 40,21.1 34.2,23.2 33.9,28.3 33.9,25.7 33.9,24.6 41.8,32.1 41.8,31.2 40.9,32.1 49.7,36.5 53.1,34.1 48.8,37.4 27.3,29.4 31.4,26.1 27.3,27.8 12.3,26.7 18.4,25.2 17.7,54.1 17.7,55 18.6,55 18.6,54.1 16.8,54.1 16.8,55 52.1,34.1 52.1,33.2 62.1,32.8 67.8,41.1 69.6,36.4 52.9,38.4 51.7,39.8 59.9,41.3 61,41.3 62.2,41 72,40.5 69.4,51 65.8,51 57.1,50.8 54.1,50.8 50.6,50.8 38,52.6 43.2,52.2 45.6,47.2 39.7,47.4 63.4,24.3 61.7,22.5 62.5,11.7 71.7,11.5 60.1,11.7 48.2,12 44.2,13.4 34.9,8.5 33.2,11.2 33.2,12.6 33.2,14.2 30.4,15.8 52.2,23.5 51.9,21.9 51.1,21.9 59.8,27.1 69.6,39 72,39.3 69.6,37.7 31.6,48.6 31.6,46.8 31.2,43.7 28.5,50.8 29.3,50.8 30.1,50.8 44.9,12 41.6,17 41.6,21.3 65.6,16.3 66.4,16.3 67.2,16.3 74.4,18.8 74.2,25.1 67.4,30.1 72,38.1 48.4,31.7 47.8,38.4 40.4,34.6 50.3,29.8 46.01,25.96 46.01,26.98 46.01,28 46.01,24.95 46.01,23.93 45,25.96 43.98,24.95 47.03,25.96 48.05,25.96 47.03,24.95 47.03,23.93 43.98,26.98 45,26.98 47.03,26.98 47.03,28 48.05,26.98 48.05,28 27.3,28.6 38.9,34.6 61,32.8 54.2,41.7 56.8,31 57.6,31.8 58.4,32.5 63,25 60.9,22.7 27.4,31.6 34.1,32.3 41.6,37 36.4,12.6 30.1,40.7 32.5,26 33.1,28.3 27.9,24.5 29.5,27 50.7,24
  pour Top (isolate 0.2): 9.8,28.8 9.8,24.3 26.3,24.3 26.3,11.3 26.8,10.8 29.8,7.8 29.8,3.8 79.8,3.8 79.8,58.3 49.8,58.3 9.8,58.3 9.8,50.95 23.8,50.95 23.8,27.8 23.3,27.3 20.3,27.3 18.8,28.8
  pour Bottom (isolate 0.2): 8.8,28.8 8.8,24.3 26.3,24.3 26.3,11.3 26.8,10.8 29.8,7.8 29.8,2.8 80.8,2.8 80.8,59.3 49.3,59.3 8.8,59.3 8.8,50.93 23.8,50.93 23.8,27.8 23.3,27.3 20.3,27.3 18.8,28.8
LINK_N  (via drill 0.3)
  Top 0.2: LED3.K 63.35,34.27 58.41,34.27 | 58.41,34.27 54.24,30.1 54.24,21.25 51.59,18.59 47.16,18.59 45.24,20.51 U1.17 | v55.4,35.4 53.37,35.4 49.14,39.63 44.41,39.63 43.48,38.7 34.4,38.7 30.49,42.61 30.49,43.8 28.41,45.88 P3.L3 | v58.4,34.3 58.41,34.29 58.41,34.27
  Bottom 0.2: v55.4,35.4 56.5,34.3 v58.4,34.3
MISO  (via drill 0.3, 0.35)
  Top 0.2: v52.14,27.48 51.46,27.48 51.14,27.16 U1.33 | P2.7 57.71,15.19 55.3,17.6 55.3,23.34 55.66,23.7 55.86,23.7 55.9,23.74 v55.9,24.3 | v67.95,32.91 67.36,33.5 v65.8,33.5 | v58,38.9 R21.2
  Bottom 0.2: v52.14,27.48 53.47,27.48 53.75,27.21 55.28,27.21 55.9,26.58 v55.9,24.3 59.4,24.3 67.8,32.7 | 67.8,32.7 69.88,34.78 JP1.1 | 67.8,32.7 67.8,32.75 v67.95,32.91 | v65.8,33.5 60.4,38.9 v58,38.9
MOSI  (via drill 0.3, 0.35)
  Top 0.2: v55.3,25.03 56.27,25.03 56.5,24.8 56.5,22.5 56.92,22.08 U5.2 | v66.5,32.8 67.2,32.8 67.34,32.66 | v67.98,32.02 67.7,32.3 67.34,32.66 | 67.34,32.66 | v58,40.4 R22.2 | U1.32 49.45,26.65 v52.31,26.65
  Bottom 0.2: v52.31,26.65 54.43,26.65 54.66,26.88 55.14,26.88 55.48,26.54 55.48,25.8 55.3,25.62 v55.3,25.03 55.3,24 55.6,23.7 56.3,23.7 56.57,23.97 59.53,23.97 67.53,31.97 67.92,31.97 v67.98,32.02 69.36,33.4 75.31,33.4 JP1.4 | v66.5,32.8 66.41,32.89 66.41,33.75 59.76,40.4 v58,40.4
MOSI3
  Top 0.2: U5.4 61.37,21.43 62.6,20.2 62.6,19.8 62.81,19.59 P2.3
N$1
  Top 0.2: LED3.A R9.1
N$2  (via drill 0.3)
  Top 0.2: 37.61,36.72 R18.2 v36.6,36.3
  Bottom 0.2: v36.6,36.3 36.6,33.5 34.6,31.5 29.2,31.5 28.05,32.65 P3.L2
N$3
  Top 0.3: R7.1 13.36,25.72 LED1.A
N$4
  Top 0.2: LED4.A R10.1
N$5
  Top 0.2: LED5.A R11.1
N$6
  Top 0.2: LED6.A R12.1
N$7
  Top 0.2: R13.1 LED7.A
N$8
  Top 0.2: R19.2 34.81,37.83 30.17,42.47 30.17,43.53 28.8,44.9 27.4,44.9 27,45.3 27,46.1 26.2,46.9 P3.L4
N$9
  Top 0.8: P3.P$4 19.95,30.3 C9.1
N$10
  Top 0.2: R3.1 R5.2
N$12
  Top 0.2: R15.2 R14.2 C27.2
N$13
  Top 0.3: U4.4 17.2,27.5 R8.2
N$14
  Top 0.3: R8.1 13.31,27.5 LED2.A
N$15
  Top 0.2: C28.2 R17.2 R16.2
N$16
  Top 0.3: R20.1 46.6,33.62 46.6,32.5 46.1,32 44.44,32 43.74,31.3 U1.47
N$17  (via drill 0.35)
  Top 0.2: v51.6,22.76 51.6,22.7 51.14,23.16 U1.25 | 57.18,13.65 JP12.1 56.27,14.56 R4.2 55.3,14.6 55.3,17.1 54.7,17.7 v54.7,20.2
  Bottom 0.2: v54.7,20.2 52.14,22.76 v51.6,22.76
N$20
  Top 0.2: R3.2 37.84,27.16 39.11,25.89 40.24,24.76 40.34,24.66 U1.9
RESET  (via drill 0.3)
  Top 0.152: SW1.3 SW1.4
  Top 0.2: C19.1 R2.1 45.1,36.68 R30.1 44.89,35.63 U3.3 | SW1.3 13.64,51.83 14.11,52.31 | 21.39,52.31 SW1.4 30.47,51.83 31.27,51.03 31.27,50.6 32.5,49.37 32.5,45.97 v32.43,45.9 | C19.1 45.02,38.38 45.28,38.38 46.2,39.3 48.91,39.3 53.41,34.8 v54.7,34.8 | v67.8,29.2 67.27,29.2 62.87,33.6 v59.1,33.6 | C19.1 43.94,38.34 v43.9,38.3
  Bottom 0.2: v32.43,45.9 33.33,45 43.4,45 43.9,44.5 v43.9,38.3 | JP1.5 73.43,29.2 v67.8,29.2 67.8,27.23 53.96,13.39 52.4,13.39 48.56,9.55 46.03,9.55 U$4.RESET | v54.7,34.8 55.9,33.6 v59.1,33.6
RESET_W
  Top 0.2: R30.2 43.72,33.64 43.56,33.48 U3.2 43.24,33.16 U1.48
RXIN
  Top 0.2: P3.6 28.05,39.66 R17.1 31.05,36.66 31.05,35.55 31.47,35.13 32.69,35.13 33.33,34.48 33.33,31.59 34.19,30.73 37.14,30.73 38.53,29.34 38.53,28.23 40.1,26.66 U1.5
RXIP
  Top 0.2: 30.16,36 30.16,35.44 30.8,34.8 32.55,34.8 33,34.35 33,31.25 33.85,30.4 37,30.4 38.2,29.2 38.2,28.1 40.14,26.16 U1.6 | 30.16,36 R16.1 | 30.16,36 29.41,36.75 27.43,36.75 P3.3
SCK3
  Top 0.2: U6.4 60.66,19.14 62.41,17.39 P2.5
SCL
  Top 0.2: 29.25,54.35 31.6,52 31.6,50.8 33.65,48.75 JP3.4 | 29.25,54.35 29.1,54.5 | U$4.SCL 29.1,54.5 | 29.1,54.5 29.25,54.35
  Bottom 0.2: JP3.4 JP2.4
SCLK  (via drill 0.3, 0.35)
  Top 0.2: v52.3,25.37 52.25,25.42 51.46,25.42 51.21,25.66 U1.30 | U6.2 56.71,19.79 55.9,20.6 v55.9,23.12 | v68,31 66.81,32.2 66.25,32.2 65.83,32.62 v65.62,32.62 | v57.77,37.73 57.44,37.4 R23.2
  Bottom 0.2: JP1.3 69.24,32.24 v68,31 | v52.3,25.37 53.47,25.37 55.72,23.12 v55.9,23.12 56.15,23.37 56.44,23.37 56.71,23.65 59.67,23.65 66.96,30.94 67.94,30.94 v68,31 | 68.21,31.21 v68,31 | v65.62,32.62 60.5,37.73 v57.77,37.73
SDA
  Top 0.2: JP3.3 36.18,47.96 36.18,49.16 35.24,50.1 32.83,50.1 31.93,51 31.93,54.81 U$4.SDA
  Bottom 0.2: JP3.3 JP2.3
SEN3
  Top 0.2: U7.4 61.78,23.72 62.5,23 62.5,21 62.81,20.69 P2.2
SPD_N
  Top 0.2: LED4.K 59.01,35.8 53.92,30.7 53.92,21.38 51.45,18.92 47.29,18.92 45.74,20.48 U1.18
TXON  (via drill 0.3)
  Top 0.2: v34.8,33.8 37.01,33.8 39.88,30.94 39.88,28.89 40.6,28.16 40.7,28.16 41.54,28.16 41.55,28.16 U1.2 | R15.1 29.53,34.43 29.53,34.44 28.23,35.73 P3.2
  Bottom 0.2: v34.8,33.8 34.75,33.8 34.38,33.43 30.53,33.43 R15.1
  other vias: 30.16,33.8
TXOP  (via drill 0.3)
  Top 0.2: v34.8,32.97 37.38,32.97 39.55,30.8 39.55,28.75 40.64,27.66 U1.3 | R14.1 29.9,32.3 29.2,33 29.2,34.3 28.78,34.73 P3.1
  Bottom 0.2: v34.8,32.97 34.67,33.1 30.96,33.1 R14.1
  other vias: 30.16,32.3
XSCI
  Top 0.2: C1.2 37.35,21.65 Y1.3 38.79,21.74 R1.1 39,22.2 39.97,23.16 U1.12
XSCO
  Top 0.2: 39.07,23.66 R1.2 38.86,23.59 | 38.86,23.59 38.07,22.8 36.5,22.8 35.66,23.64 Y1.1 35.66,25.55 C2.2 | U1.11 38.94,23.66 38.86,23.59

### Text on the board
tNames: JP11 | JP10 | JP12 | Y1 | JP8 | JP9
tSILK: RESET | SCL | SDA | AREF | GND | 13 | 12 | 11 | 10 | 9 | 8 | 7 | 6 | 5 | 4 | 3 | 2 | 1 | 0 | OUT6 | OUT5 | IN2 | IN3 | COLn | TWI | TWI | ACTn | DPXn | SPDn | LINKn | 37 | W5100S Ethernet Shield | 1 | L | ON | 25 | 13 | IOREF | RESET | 3.3V | 5V | GND | GND | Vin | A0 | A1 | A2 | A3 | A4 | A5
bSILK: TX | RX | W5100S Ethernet Shield | OPEN-SOURCE ELECTRONICS | PROTOTYPING PLATFORM | http://wiznet.io | MADE IN KOREA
